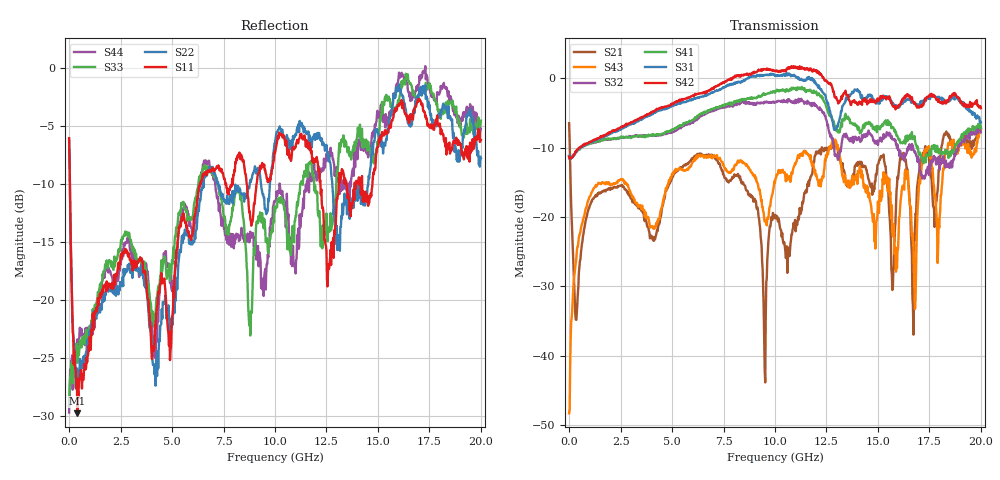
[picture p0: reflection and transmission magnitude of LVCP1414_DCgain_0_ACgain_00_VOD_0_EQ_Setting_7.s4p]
!Agilent Technologies,N5230A,MY46400459,A.07.50.48
!Agilent N5230A: A.07.50.48
!Date: Tuesday, April 17, 2012 18:35:33
!Correction: S11(Full 4 Port(1,2,3,4))
!S12(Full 4 Port(1,2,3,4))
!S13(Full 4 Port(1,2,3,4))
!S14(Full 4 Port(1,2,3,4))
!S21(Full 4 Port(1,2,3,4))
!S22(Full 4 Port(1,2,3,4))
!S23(Full 4 Port(1,2,3,4))
!S24(Full 4 Port(1,2,3,4))
!S31(Full 4 Port(1,2,3,4))
!S32(Full 4 Port(1,2,3,4))
!S33(Full 4 Port(1,2,3,4))
!S34(Full 4 Port(1,2,3,4))
!S41(Full 4 Port(1,2,3,4))
!S42(Full 4 Port(1,2,3,4))
!S43(Full 4 Port(1,2,3,4))
!S44(Full 4 Port(1,2,3,4))
!S4P File: Measurements: <S11,S12,S13,S14>,
!<S21,S22,S23,S24>,
!<S31,S32,S33,S34>,
!<S41,S42,S43,S44>:
# Hz S  dB  R 50
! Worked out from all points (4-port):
!   801 points, 300 kHz to 20 GHz, reference 50 ohm
!   strongest paths, dB at 300 kHz, 5 GHz, 10 GHz, 15 GHz, 20 GHz:
!     S42: -11.3, -3.6, 1.0, -2.9, -4.3
!     S31: -11.2, -4.0, 0.3, -3.6, -6.4
!     S41: -11.2, -7.4, -2.1, -6.9, -7.2
!     S32: -11.3, -7.8, -3.5, -9.6, -7.8
!     S43: -48.3, -13.8, -15.1, -17.8, -7.5
!     S21: -6.5, -14.3, -20.2, -12.4, -7.2
!   lowest |S11| = -29.8 dB at 400.3 MHz (marker M1), VSWR 1.07, Z = 53 + j1.43 ohm
!   |S11| at or under -10 dB: 37.59 MHz to 6.369 GHz (6.331 GHz wide, 198 % of centre); 8.623 GHz to 9.108 GHz (484.1 MHz wide, 5.46 % of centre); 12.21 GHz to 13.1 GHz (893.9 MHz wide, 7.06 % of centre)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
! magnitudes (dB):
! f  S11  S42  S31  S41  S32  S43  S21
! 300 kHz  -6.1  -11.3  -11.2  -11.2  -11.3  -48.3  -6.5
! 400.3 MHz  -29.8  -10.3  -10.3  -10.4  -10.4  -24.3  -32.3
! 10.03 GHz  -7.1  1.1  0.4  -1.9  -3.5  -14.5  -19.7
! 12.75 GHz  -15.0  -1.0  -5.7  -5.5  -8.5  -9.5  -10.1
! 16.8 GHz  -3.4  -3.5  -3.6  -9.0  -10.6  -33.3  -21.7
! 17.38 GHz  -4.4  -2.7  -2.7  -11.1  -13.7  -10.5  -10.7
! 20 GHz  -6.2  -4.3  -6.4  -7.2  -7.8  -7.5  -7.2
